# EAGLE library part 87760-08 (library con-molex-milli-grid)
HEADER
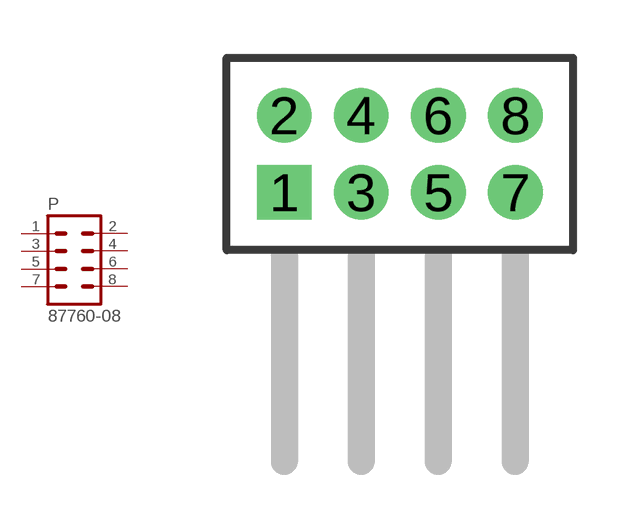
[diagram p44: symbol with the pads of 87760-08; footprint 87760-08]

Designator prefix P

## 87760-08  [87760-08]
1  1  pas
2  2  pas
3  3  pas
4  4  pas
5  5  pas
6  6  pas
7  7  pas
8  8  pas

## Footprint 87760-08 (pad centres in mm)
HEADER Dual Row, Right Angle
drill 0.914 square: 1 -3,-1
drill 0.914: 2 -3,1; 3 -1,-1; 4 -1,1; 5 1,-1; 6 1,1; 7 3,-1; 8 3,1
